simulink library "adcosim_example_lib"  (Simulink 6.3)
undefined symbols (not defined in the file or in its folder): no_bitstream
libraries: xbsIndex_r4 x6, adcosim_example_lib x1

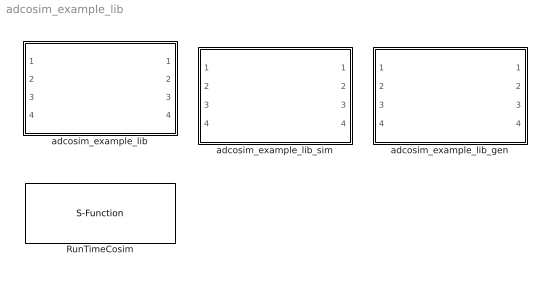
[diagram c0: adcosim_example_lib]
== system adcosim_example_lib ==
  RunTimeCosim : S-Function  FunctionName=adcosim  Parameters='enable,in,boolean,1,0;count,out,unsigned,8,0;sine,out,signed,16,0;',index,bitstream,freq,single_step,shared  mask{index=0, bitstream=no_bitstream, freq=50, single_step=off, shared=None}
      mask prompts: index "Card Index"; freq "Clock Frequency"; single_step "Single Step"; shared "Share Access"
  adcosim_example_lib : Subsystem  Tag=configX  BlockChoice=adcosim_example_lib_sim
  adcosim_example_lib_gen : Subsystem
  adcosim_example_lib_sim : Subsystem

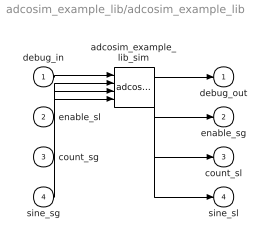
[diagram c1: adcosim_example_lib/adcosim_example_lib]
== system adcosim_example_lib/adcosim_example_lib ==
  debug_in : Inport
  enable_sl : Inport  Port=2
  count_sg : Inport  Port=3
  sine_sg : Inport  Port=4
  adcosim_example_lib_sim : adcosim_example_lib/adcosim_example_lib_sim
  debug_out : Outport
  enable_sg : Outport  Port=2
  count_sl : Outport  Port=3
  sine_sl : Outport  Port=4
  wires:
  debug_in/1 -> adcosim_example_lib_sim/1
  enable_sl/1 -> adcosim_example_lib_sim/2
  count_sg/1 -> adcosim_example_lib_sim/3
  sine_sg/1 -> adcosim_example_lib_sim/4
  adcosim_example_lib_sim/1 -> debug_out/1
  adcosim_example_lib_sim/2 -> enable_sg/1
  adcosim_example_lib_sim/3 -> count_sl/1
  adcosim_example_lib_sim/4 -> sine_sl/1

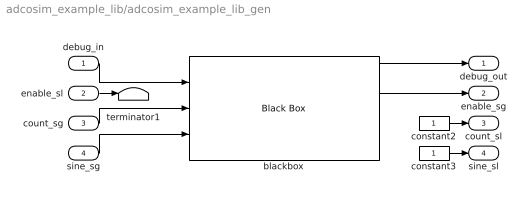
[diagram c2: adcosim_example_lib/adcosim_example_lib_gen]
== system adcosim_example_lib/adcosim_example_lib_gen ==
  debug_in : Inport
  enable_sl : Inport  Port=2
  count_sg : Inport  Port=3
  sine_sg : Inport  Port=4
  blackbox : xbsIndex_r4/Black Box  init_code=adcosim_example_lib_config  sim_method=Inactive  block_type=blackbox2
  constant2 : Constant
  constant3 : Constant
  terminator1 : Terminator
  debug_out : Outport
  enable_sg : Outport  Port=2
  count_sl : Outport  Port=3
  sine_sl : Outport  Port=4
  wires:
  enable_sl/1 -> terminator1/1
  constant2/1 -> count_sl/1
  constant3/1 -> sine_sl/1
  debug_in/1 -> blackbox/1
  blackbox/1 -> debug_out/1
  blackbox/2 -> enable_sg/1
  count_sg/1 -> blackbox/2
  sine_sg/1 -> blackbox/3

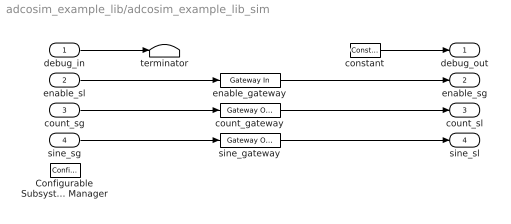
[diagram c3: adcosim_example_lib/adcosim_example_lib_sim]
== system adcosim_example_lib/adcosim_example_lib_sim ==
  debug_in : Inport
  enable_sl : Inport  Port=2
  count_sg : Inport  Port=3
  sine_sg : Inport  Port=4
  Configurable Subsystem Manager : xbsIndex_r4/Configurable Subsystem Manager  Tag=xcfgMgr  block_type=configsubsys
  constant : xbsIndex_r4/Constant  arith_type=Unsigned  const=1  n_bits=32  bin_pt=0  explicit_period=on  period=1  equ=P=C  opselect=C  inp2=PCIN>>17  opr=+  inp1=P  carry=CIN  dbl_ovrd=off  block_type=constant
  count_gateway : xbsIndex_r4/Gateway Out  hdl_port=on  timing_constraint=None  locs_specified=off  LOCs={}  block_type=gatewayout
  enable_gateway : xbsIndex_r4/Gateway In  arith_type=Boolean  n_bits=1  bin_pt=0  period=1  dbl_ovrd=off  timing_constraint=None  locs_specified=off  LOCs={}  block_type=gatewayin
  sine_gateway : xbsIndex_r4/Gateway Out  hdl_port=on  timing_constraint=None  locs_specified=off  LOCs={}  block_type=gatewayout
  terminator : Terminator
  debug_out : Outport
  enable_sg : Outport  Port=2
  count_sl : Outport  Port=3
  sine_sl : Outport  Port=4
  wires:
  debug_in/1 -> terminator/1
  constant/1 -> debug_out/1
  enable_sl/1 -> enable_gateway/1
  enable_gateway/1 -> enable_sg/1
  count_sg/1 -> count_gateway/1
  count_gateway/1 -> count_sl/1
  sine_sg/1 -> sine_gateway/1
  sine_gateway/1 -> sine_sl/1
